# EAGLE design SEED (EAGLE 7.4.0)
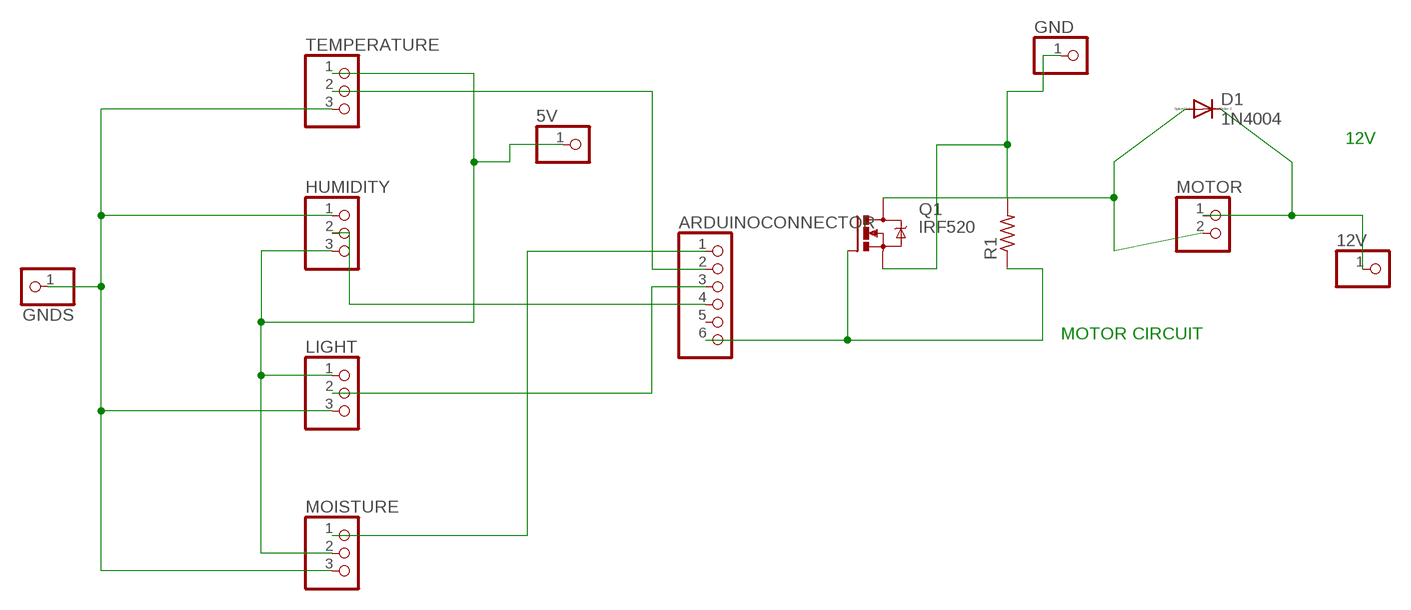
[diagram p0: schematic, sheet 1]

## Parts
5V  PINHD-1X1  [1X01]
12V  PINHD-1X1  [1X01]
ARDUINOCONNECTOR  PINHD-1X6  [1X06]
D1  1N4004  [DO41-10]
GND  PINHD-1X1  [1X01]
GNDS  PINHD-1X1  [1X01]
HUMIDITY  PINHD-1X3  [1X03]
LIGHT  PINHD-1X3  [1X03]
MOISTURE  PINHD-1X3  [1X03]
MOTOR  PINHD-1X2  [1X02]
Q1  IRF520  [TO220BV]
R1  R-US_0207/12  [0207/12]
TEMPERATURE  PINHD-1X3  [1X03]

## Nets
N$1: ARDUINOCONNECTOR.1 MOISTURE.1
N$2: ARDUINOCONNECTOR.2 TEMPERATURE.2
N$3: ARDUINOCONNECTOR.3 LIGHT.2
N$4: ARDUINOCONNECTOR.4 HUMIDITY.2
N$5: ARDUINOCONNECTOR.6 Q1.G R1.1
N$7: D1.A MOTOR.2 Q1.D
N$8: 5V.1 HUMIDITY.3 LIGHT.1 MOISTURE.2 TEMPERATURE.1
N$9: 12V.1 D1.C MOTOR.1
N$10: GND.1 Q1.S R1.2
N$11: GNDS.1 HUMIDITY.1 LIGHT.3 MOISTURE.3 TEMPERATURE.3
Unconnected: ARDUINOCONNECTOR.5

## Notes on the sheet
- 12V
- MOTOR CIRCUIT

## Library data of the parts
5V 12V GND GNDS = pinhead:PINHD-1X1: PIN HEADER
ARDUINOCONNECTOR = pinhead:PINHD-1X6: PIN HEADER
D1 = diode:1N4004: DIODE
HUMIDITY LIGHT MOISTURE TEMPERATURE = pinhead:PINHD-1X3: PIN HEADER
MOTOR = pinhead:PINHD-1X2: PIN HEADER
Q1 = transistor-power:IRF520: HEXFET Power MOSFET
R1 = resistor:R-US_: RESISTOR, American symbol

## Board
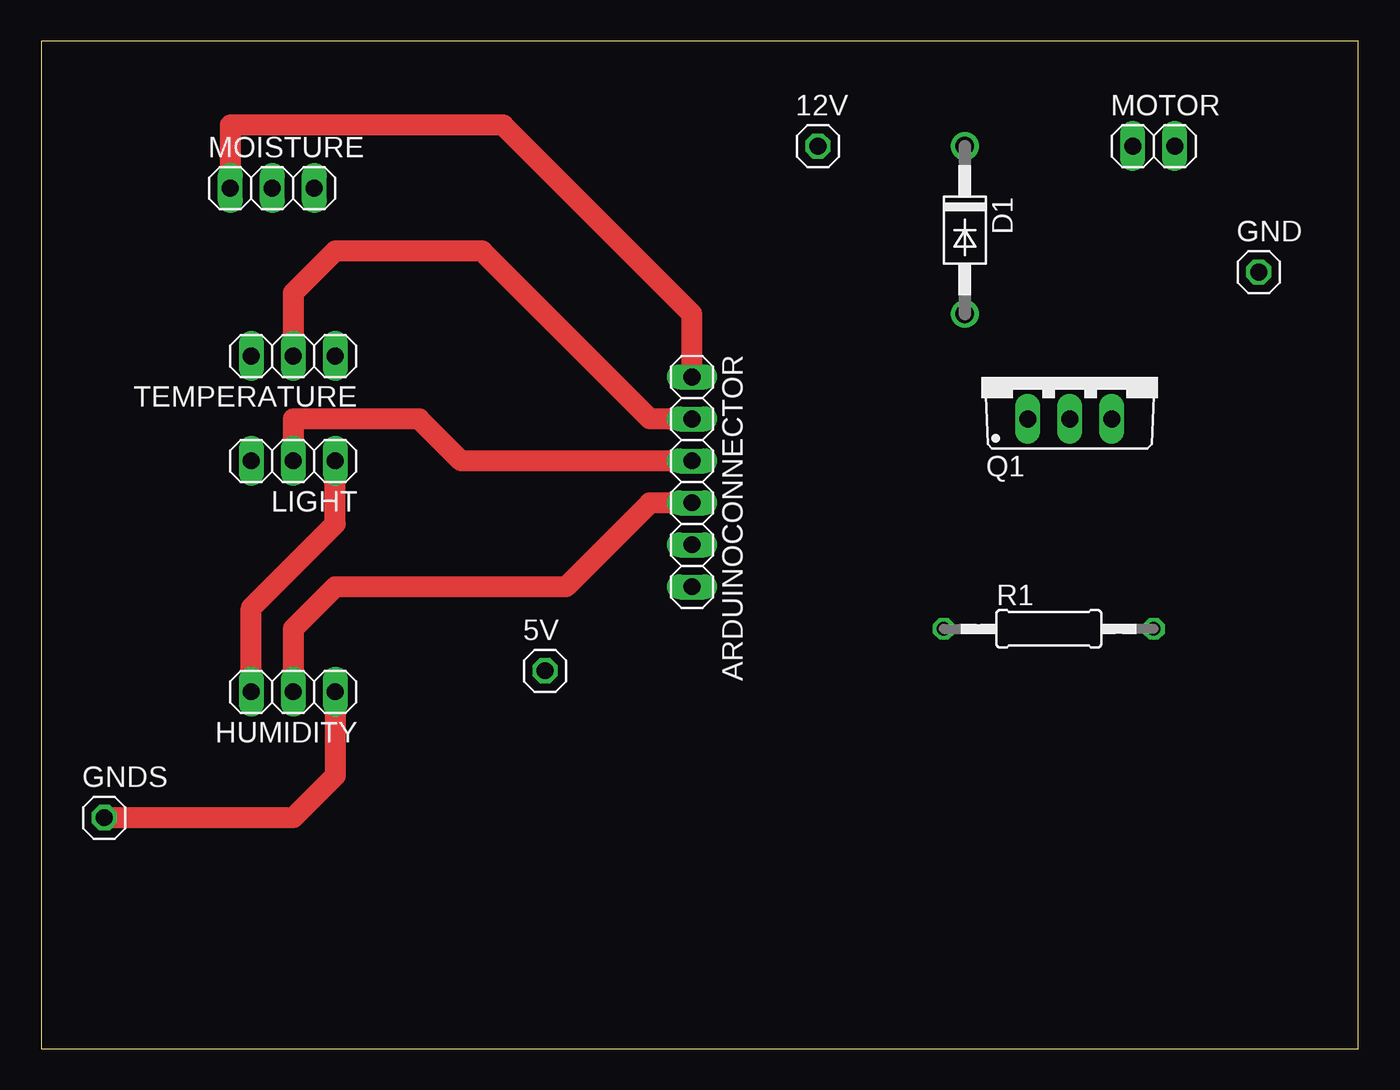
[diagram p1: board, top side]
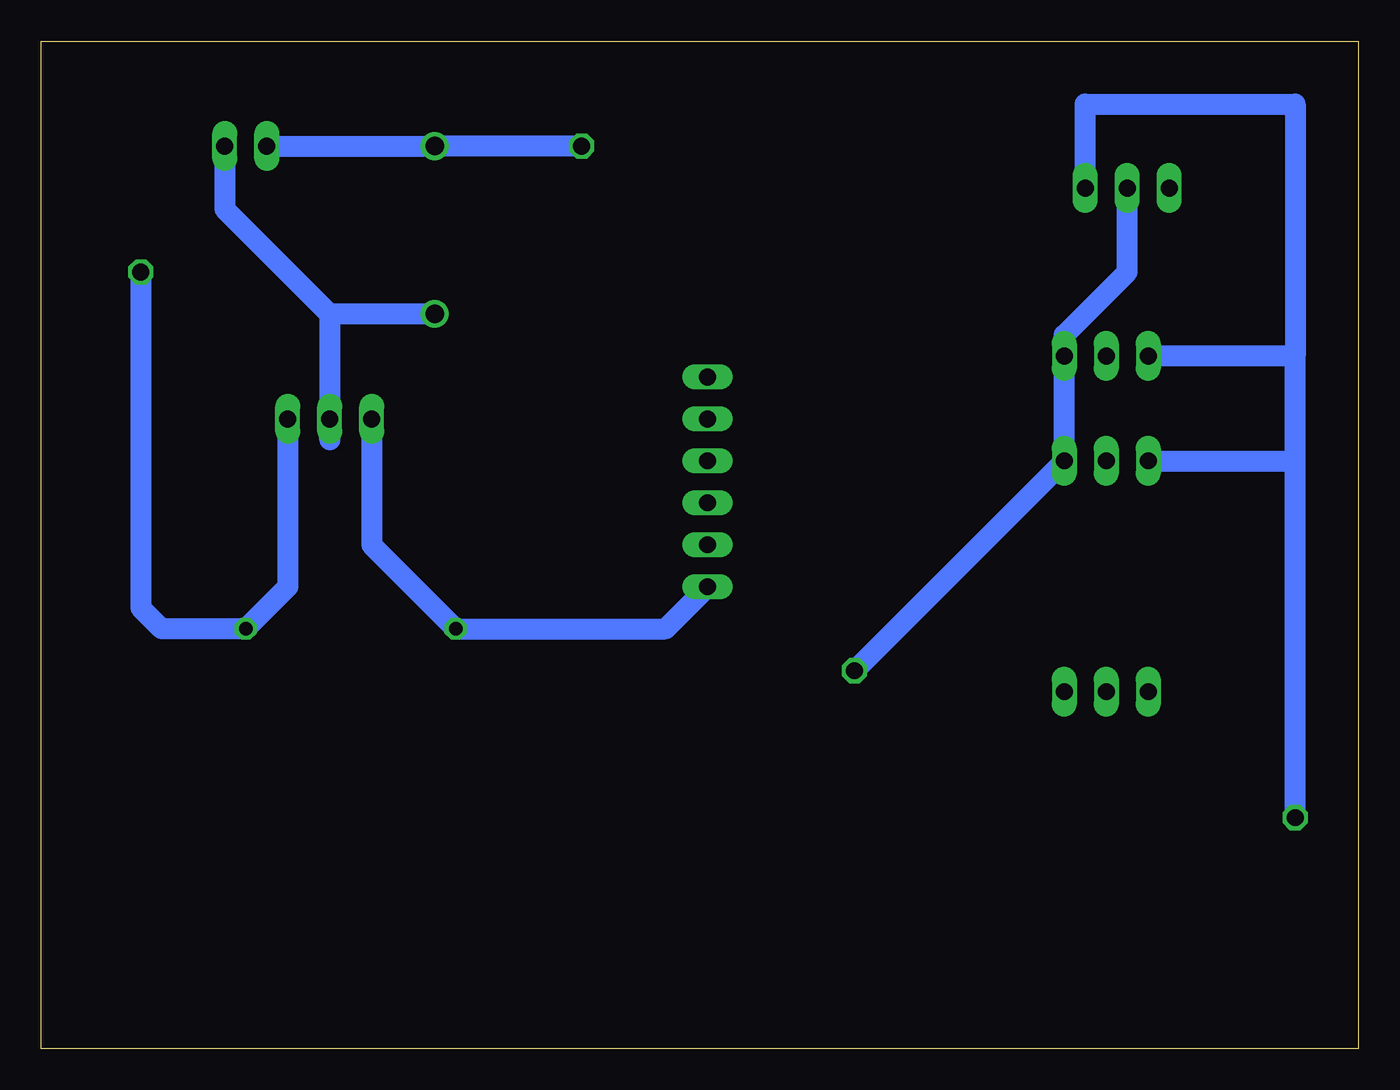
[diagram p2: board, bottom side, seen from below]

Size 79.68 x 60.95 mm. Coordinates in mm from the lower left corner, seen from the top.
Outline: 0,0 79.68,0 79.68,60.95 0,60.95 0,0
Copper layers (1*16): Top 0.035mm / dielectric 1.5mm / Bottom 0.035mm
Design rules "default": minimum track width 10mil, minimum drill 24mil, track to track 8mil, track to pad 8mil, pad to pad 8mil, via to via 8mil, smd to smd 8mil, copper to edge 40mil, drill to drill 8mil, minimum pad ring 10mil, minimum via ring 8mil, stop-mask expansion 4mil, vias tented up to drill 0mil, thermal gap 10mil

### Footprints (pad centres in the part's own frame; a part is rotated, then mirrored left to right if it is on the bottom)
1X01 = drill 1.016 octagon: 1 0,0
1X06 = drill 1.016 long: 1 -6.35,0; 2 -3.81,0; 3 -1.27,0; 4 1.27,0; 5 3.81,0; 6 6.35,0
DO41-10 = drill 1.118: A 5.08,0; C -5.08,0
1X03 = drill 1.016 long: 1 -2.54,0; 2 0,0; 3 2.54,0
1X02 = drill 1.016 long: 1 -1.27,0; 2 1.27,0
TO220BV = drill 1.016 long: D 0,-2.54; G -2.54,-2.54; S 2.54,-2.54
0207/12 = drill 0.813 octagon: 1 -6.35,0; 2 6.35,0

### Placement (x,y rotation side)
5V  30.48,22.86 0 top
12V  46.99,54.61 0 top
ARDUINOCONNECTOR  39.37,34.29 270 top
D1  55.88,49.53 270 top
GND  73.66,46.99 0 top
GNDS  3.81,13.97 0 top
HUMIDITY  15.24,21.59 180 top
LIGHT  15.24,35.56 180 top
MOISTURE  13.97,52.07 0 top
MOTOR  67.31,54.61 0 top
Q1  62.23,40.64 0 top
R1  60.96,25.4 0 top
TEMPERATURE  15.24,41.91 180 top

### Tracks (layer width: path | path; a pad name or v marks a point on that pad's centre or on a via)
N$1
  Top 1.27: ARDUINOCONNECTOR.1 39.37,44.45 27.94,55.88 11.43,55.88 MOISTURE.1
N$2
  Top 1.27: ARDUINOCONNECTOR.2 36.83,38.1 26.67,48.26 17.78,48.26 15.24,45.72 TEMPERATURE.2
N$3
  Top 1.27: ARDUINOCONNECTOR.3 25.4,35.56 22.86,38.1 15.24,38.1 LIGHT.2
N$4
  Top 1.27: ARDUINOCONNECTOR.4 36.83,33.02 31.75,27.94 17.78,27.94 15.24,25.4 HUMIDITY.2
N$5
  Bottom 1.27: Q1.G 59.69,30.48 R1.1 41.91,25.4 ARDUINOCONNECTOR.6
N$7
  Bottom 1.27: MOTOR.2 68.58,50.8 62.23,44.45 | 62.23,44.45 Q1.D 62.23,36.83 | D1.A 62.23,44.45
N$8
  Top 1.27: HUMIDITY.3 12.7,26.67 17.78,31.75 LIGHT.1
  Bottom 1.27: MOISTURE.2 13.97,46.99 17.78,43.18 TEMPERATURE.1 LIGHT.1 5V.1
N$9
  Bottom 1.27: 12V.1 D1.C MOTOR.1
N$10
  Bottom 1.27: Q1.S 64.77,27.94 R1.2 72.39,25.4 73.66,26.67 GND.1
N$11
  Top 1.27: HUMIDITY.1 17.78,16.51 15.24,13.97 GNDS.1
  Bottom 1.27: GNDS.1 3.81,35.56 | 3.81,35.56 3.81,41.91 | 3.81,41.91 TEMPERATURE.3 | LIGHT.3 3.81,35.56 | MOISTURE.3 16.51,57.15 3.81,57.15 3.81,41.91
